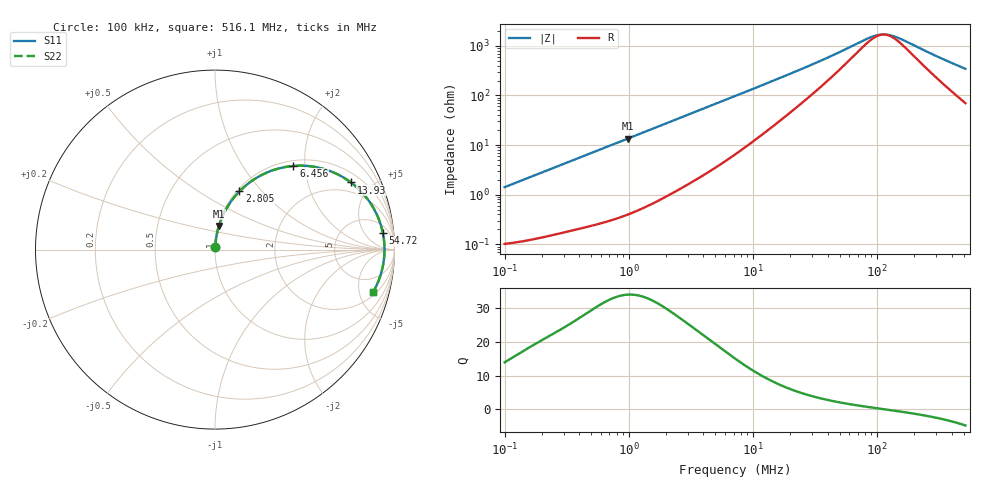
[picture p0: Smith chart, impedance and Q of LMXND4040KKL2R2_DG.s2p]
! LMXND4040KKL2R2_DG  S-PARAMETER MODEL  ( General Type )
! Model Generated by TAIYO YUDEN Corporation (http://www.ty-top.com)
! Version 1.0
! TAIYO YUDEN Control No. 191023NI43SB-FBB
! Copyright(c) 2019 TAIYO YUDEN CO.,LTD. All Rights Reserved.
! Product Description (link to TY-COMPAS)
! https://ds.yuden.co.jp/TYCOMPAS/or/detail?pn=LMXND4040KKL2R2MDG&u=M
! Products Name : Inductors
! Characteristics :
!  Inductance : 2.2 uH , SRF(min) : 73 MHz , DC Resistance(max) : 0.102 Ohm
!  Rated Current : Saturation :1200 mA , Temp Rise : 1500 mA
!  Case Size : 4.0 x 4.0 / 0.157 x 0.157 [mm/inch] , Thickness : 1 / 0.039 [mm/inch]
!  (Conditions: Temperature = 25 degC , DC Bias Current/Voltage = 0A / 0V)
! External Node Assignments :
!  1  o---GGG---o  2
! GND o---------o GND
! Frequency Range : 0.1MHz  -  516.089782MHz  [ 402 STEP ]
# MHz S RI R 50
! Freq[MHz].  S11 Real  S11 Imag  S21 Real  S21 Imag  S12 Real  S12 Imag  S22 Real  S22 Imag
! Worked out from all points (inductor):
!   401 points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, 100 kHz to 516.1 MHz, reference 50 ohm
!   read as one part in series: L = 2.25 uH near 104.4 kHz
!   highest Q = 34 at 984.4 kHz (marker M1), where L = 2.19 uH
!   self-resonance near 113.4 MHz
!   S11 on the Smith chart (normalised r, x): 100 kHz: 1.00, +0.03; 2.805 MHz: 1.03, +0.76; 6.456 MHz: 1.11, +1.74; 13.93 MHz: 1.44, +3.76; 54.72 MHz: 9, +15; 516.1 MHz: 2.40, -6.75
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0.1  0.00122 0.0141  0.9988 -0.0141  0.9988 -0.0141  0.00122 0.0141
0.220509  0.0024 0.0308  0.9976 -0.0308  0.9976 -0.0308  0.0024 0.0308
0.418679  0.00545 0.0577  0.9946 -0.0577  0.9946 -0.0577  0.00545 0.0577
0.98436  0.0217 0.1318  0.9783 -0.1318  0.9783 -0.1318  0.0217 0.1318
1.752923  0.0607 0.2233  0.9393 -0.2233  0.9393 -0.2233  0.0607 0.2233
2.805194  0.1365 0.3247  0.8635 -0.3247  0.8635 -0.3247  0.1365 0.3247
4.121312  0.2479 0.4093  0.7521 -0.4093  0.7521 -0.4093  0.2479 0.4093
5.213573  0.3405 0.448  0.6595 -0.448  0.6595 -0.448  0.3405 0.448
6.455852  0.4366 0.4662  0.5634 -0.4662  0.5634 -0.4662  0.4366 0.4662
7.183939  0.4866 0.4677  0.5134 -0.4677  0.5134 -0.4677  0.4866 0.4677
9.689648  0.6225 0.4443  0.3775 -0.4443  0.3775 -0.4443  0.6225 0.4443
13.93474  0.7572 0.3741  0.2428 -0.3741  0.2428 -0.3741  0.7572 0.3741
20.03963  0.8463 0.2865  0.1537 -0.2865  0.1537 -0.2865  0.8463 0.2865
30.07766  0.9016 0.1953  0.0984 -0.1953  0.0984 -0.1953  0.9016 0.1953
54.71859  0.9353 0.0919  0.0647 -0.0919  0.0647 -0.0919  0.9353 0.0919
78.69112  0.9424 0.0435  0.0576 -0.0435  0.0576 -0.0435  0.9424 0.0435
93.36416  0.9438 0.0228  0.0562 -0.0228  0.0562 -0.0228  0.9438 0.0228
108.4309  0.9444 0.0052  0.0556 -0.0052  0.0556 -0.0052  0.9444 0.0052
125.929  0.9443 -0.0123  0.0557 0.0123  0.0557 0.0123  0.9443 -0.0123
152.6377  0.9431 -0.0352  0.0569 0.0352  0.0569 0.0352  0.9431 -0.0352
309.0023  0.9247 -0.135  0.0753 0.135  0.0753 0.135  0.9247 -0.135
516.0898  0.881 -0.2362  0.119 0.2362  0.119 0.2362  0.881 -0.2362
